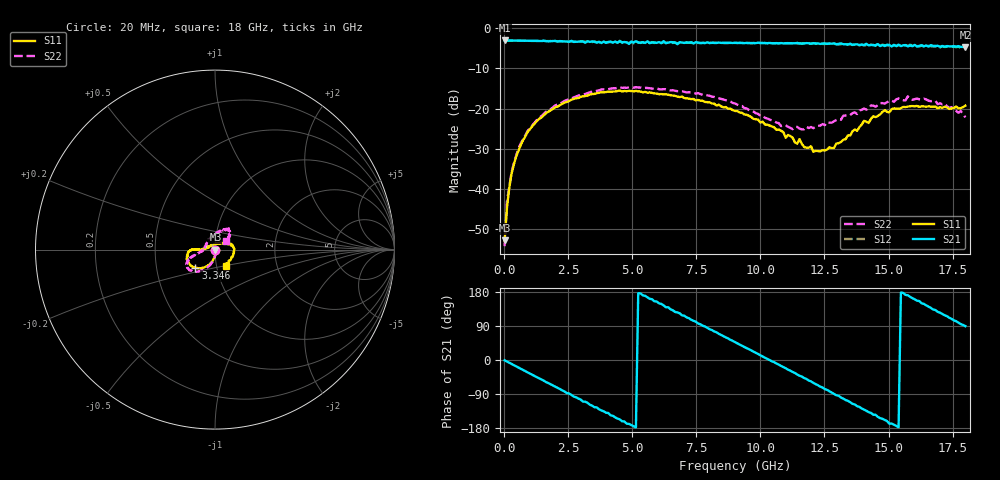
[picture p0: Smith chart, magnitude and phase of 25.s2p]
!Agilent Technologies,N5230A,US43500223,A.07.50.48
!Agilent N5230A: A.07.50.48
!Date: Saturday, January 16, 2016 11:05:13
!Correction: S11(Full 2 Port(1,2))
!S21(Full 2 Port(1,2))
!S12(Full 2 Port(1,2))
!S22(Full 2 Port(1,2))
!S2P File: Measurements: S11, S21, S12, S22:
# Hz S  dB  R 50
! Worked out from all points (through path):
!   201 points, 20 MHz to 18 GHz, reference 50 ohm
!   highest |S21| = -3.02 dB at 20 MHz (marker M1); lowest = -4.7 dB at 18 GHz (marker M2)
!   group delay of S21, straight-line fit = 97.1 ps
!   lowest |S11| = -52.9 dB at 20 MHz (marker M3), VSWR 1.00, Z = 50.2 - j0.0243 ohm
!   |S11| at or under -10 dB: start of sweep to end of sweep
!   |S22| runs from -54.3 to -14.7 dB; largest |S21 - S12| = 0.054
!   S11 on the Smith chart (normalised r, x): 20 MHz: 1.00, -0.00; 3.346 GHz: 0.79, -0.16; 18 GHz: 1.11, -0.20
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2e7  -52.91 -6.1  -3.02 -0.8  -3.01 -0.8  -54.34 -14.5
1.099e8  -44.90 -60.3  -3.03 -4.0  -3.02 -4.2  -43.29 -56.2
2.897e8  -36.31 -75.8  -3.04 -10.4  -3.04 -10.6  -36.00 -77.3
6.493e8  -29.10 -90.7  -3.07 -23.2  -3.07 -23.3  -28.69 -90.0
1.818e9  -20.45 -113.7  -3.18 -64.2  -3.14 -65.0  -20.16 -110.4
3.0766e9  -16.94 -133.5  -3.25 -109.8  -3.27 -109.2  -16.50 -126.7
3.3463e9  -16.54 -137.1  -3.37 -118.0  -3.44 -119.1  -15.92 -129.7
4.515e9  -15.48 -154.0  -3.22 -156.8  -3.09 -157.9  -14.68 -141.7
5.1443e9  -15.61 -161.6  -3.20 -178.0  -3.12 -179.0  -14.67 -147.7
6.0433e9  -16.42 -172.2  -3.42 149.6  -3.51 147.4  -15.19 -153.0
7.4817e9  -17.97 -179.8  -3.43 101.1  -3.61 98.6  -16.26 -158.8
8.2009e9  -18.78 -179.1  -3.63 75.3  -3.57 73.9  -17.11 -161.3
9.01e9  -20.59 179.3  -3.58 47.2  -3.63 45.4  -18.72 -164.6
9.909e9  -22.75 179.3  -3.58 15.9  -3.67 13.9  -21.33 -169.5
1.06282e10  -25.31 175.8  -3.67 -9.4  -3.69 -11.2  -23.51 -175.1
1.20666e10  -30.79 128.3  -3.68 -60.3  -3.73 -62.5  -24.90 138.6
1.3505e10  -26.74 49.1  -3.82 -111.4  -3.95 -113.8  -21.64 92.4
1.40444e10  -23.06 32.5  -4.13 -130.9  -4.30 -132.9  -20.00 81.3
1.50333e10  -20.94 16.4  -4.14 -168.0  -4.36 -168.8  -18.08 66.6
1.62919e10  -19.43 -6.4  -4.21 149.7  -4.23 147.4  -17.74 52.0
1.69212e10  -19.95 -24.1  -4.34 126.9  -4.43 123.2  -18.90 47.5
1.8e10  -19.28 -56.1  -4.70 89.3  -4.70 84.8  -22.20 36.4
